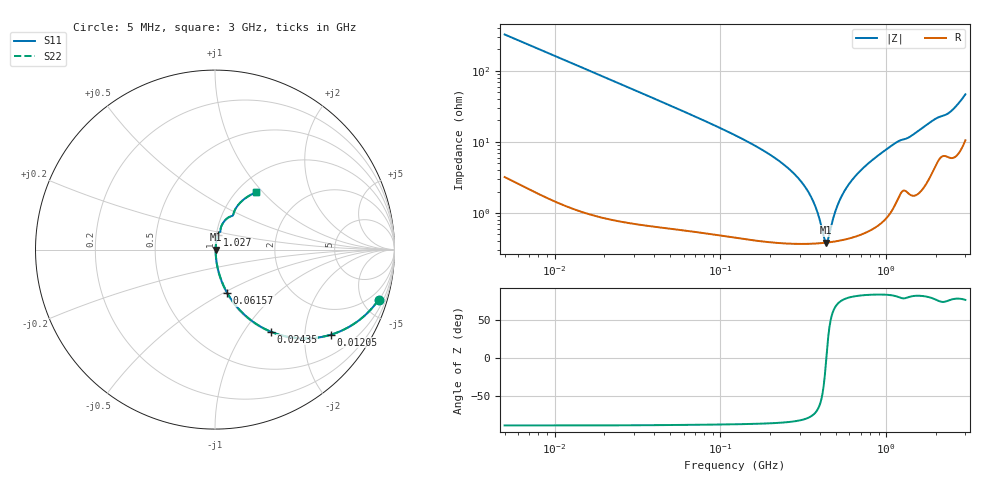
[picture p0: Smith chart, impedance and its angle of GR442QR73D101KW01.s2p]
!Murata Part Number: GR442QR73D101KW01
!These Parameters are Measured in Series Mode Connection
!Data Generated on Mar 13, 2026
!  o--ll--o
!Port1  Port2
!  o------o
!Operation Temp=25[degC], DC Bias Voltage=0[V]
!Freq. Start=5[MHz] Stop=3[GHz] 401[Steps]
# Hz S RI R 50
!Freq.(Hz) S11(Real) S11(Imag) S21(Real) S21(Imag) S12(Real) S12(Imag) S22(Real) S22(Imag)
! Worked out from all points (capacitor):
!   401 points, 5 MHz to 3 GHz, reference 50 ohm
!   read as one part in series: C = 97.9 pF near 5.163 MHz
!   lowest |Z| = 384 mohm at 433.2 MHz (marker M1)
!   series resonance near 435.2 MHz, so ESL is about 1.4 nH
!   S11 on the Smith chart (normalised r, x): 5 MHz: 1.06, -6.49; 12.05 MHz: 1.02, -2.70; 24.35 MHz: 1.02, -1.34; 61.57 MHz: 1.01, -0.52; 1.027 GHz: 1.02, +0.16; 3 GHz: 1.21, +0.91
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5000000  0.9111 -0.2798  0.0889 0.2798  0.0889 0.2798  0.9111 -0.2798
7824212  0.81 -0.3877  0.19 0.3877  0.19 0.3877  0.81 -0.3877
1.204941e7  0.6451 -0.474  0.3549 0.474  0.3549 0.474  0.6451 -0.474
1.459857e7  0.5542 -0.4924  0.4458 0.4924  0.4458 0.4924  0.5542 -0.4924
2.435356e7  0.3109 -0.4572  0.6891 0.4572  0.6891 0.4572  0.3109 -0.4572
4.262365e7  0.1304 -0.3286  0.8696 0.3286  0.8696 0.3286  0.1304 -0.3286
6.157358e7  0.0684 -0.2419  0.9316 0.2419  0.9316 0.2419  0.0684 -0.2419
1.244489e8  0.0189 -0.1191  0.9811 0.1191  0.9811 0.1191  0.0189 -0.1191
2.475382e8  0.00575 -0.0451  0.9942 0.0451  0.9942 0.0451  0.00575 -0.0451
3.047419e8  0.00443 -0.0277  0.9956 0.0277  0.9956 0.0277  0.00443 -0.0277
3.575905e8  0.00391 -0.0151  0.9961 0.0151  0.9961 0.0151  0.00391 -0.0151
3.873583e8  0.0038 -0.00894  0.9962 0.00894  0.9962 0.00894  0.0038 -0.00894
4.196041e8  0.00378 -0.0028  0.9962 0.0028  0.9962 0.0028  0.00378 -0.0028
4.33242e8  0.00381 -0.000344  0.9962 0.000344  0.9962 0.000344  0.00381 -0.000344
4.47323e8  0.00384 0.00212  0.9962 -0.00212  0.9962 -0.00212  0.00384 0.00212
5.083751e8  0.00416 0.0121  0.9958 -0.0121  0.9958 -0.0121  0.00416 0.0121
5.870738e8  0.00487 0.0236  0.9951 -0.0236  0.9951 -0.0236  0.00487 0.0236
7.343921e8  0.007 0.0432  0.993 -0.0432  0.993 -0.0432  0.007 0.0432
1.027498e9  0.0154 0.0795  0.9846 -0.0795  0.9846 -0.0795  0.0154 0.0795
1.044062e9  0.0162 0.0815  0.9838 -0.0815  0.9838 -0.0815  0.0162 0.0815
2.436864e9  0.1093 0.2177  0.8907 -0.2177  0.8907 -0.2177  0.1093 0.2177
3e9  0.2264 0.3185  0.7736 -0.3185  0.7736 -0.3185  0.2264 0.3185
